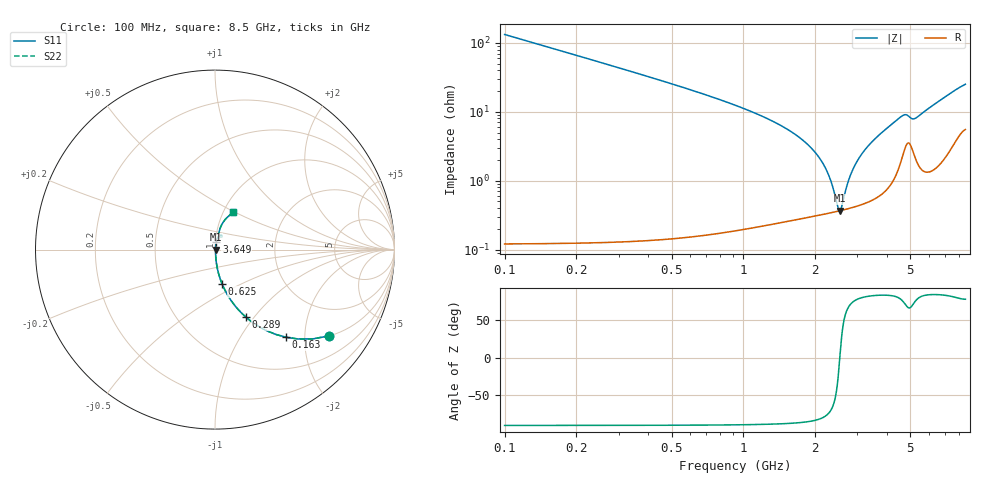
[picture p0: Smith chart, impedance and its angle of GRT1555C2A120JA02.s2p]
!Murata Part Number: GRT1555C2A120JA02
!These Parameters are Measured in Series Mode Connection
!Data Generated on Jun 19, 2026
!  o--ll--o
!Port1  Port2
!  o------o
!Operation Temp=25[degC], DC Bias Voltage=0[V]
!Freq. Start=100[MHz] Stop=9[GHz] 401[Steps]
# Hz S RI R 50
!Freq.(Hz) S11(Real) S11(Imag) S21(Real) S21(Imag) S12(Real) S12(Imag) S22(Real) S22(Imag)
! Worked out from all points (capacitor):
!   401 points, 100 MHz to 8.5 GHz, reference 50 ohm
!   read as one part in series: C = 12 pF near 142 MHz
!   lowest |Z| = 367 mohm at 2.536 GHz (marker M1)
!   series resonance near 2.532 GHz, so ESL is about 330 pH
!   S11 on the Smith chart (normalised r, x): 100 MHz: 1.00, -2.65; 163 MHz: 1.00, -1.62; 289 MHz: 1.00, -0.91; 625 MHz: 1.00, -0.40; 3.649 GHz: 1.01, +0.09; 8.5 GHz: 1.11, +0.49
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1e8  0.6367 -0.4805  0.3633 0.4805  0.3633 0.4805  0.6367 -0.4805
1.63e8  0.3965 -0.4884  0.6035 0.4884  0.6035 0.4884  0.3965 -0.4884
2.89e8  0.1709 -0.375  0.8291 0.375  0.8291 0.375  0.1709 -0.375
4.15e8  0.0892 -0.2829  0.9108 0.2829  0.9108 0.2829  0.0892 -0.2829
6.25e8  0.0396 -0.1911  0.9604 0.1911  0.9604 0.1911  0.0396 -0.1911
1.507e9  0.00578 -0.0568  0.9942 0.0568  0.9942 0.0568  0.00578 -0.0568
1.885e9  0.00395 -0.0317  0.996 0.0317  0.996 0.0317  0.00395 -0.0317
2.137e9  0.00354 -0.0182  0.9965 0.0182  0.9965 0.0182  0.00354 -0.0182
2.284e9  0.00349 -0.0111  0.9965 0.0111  0.9965 0.0111  0.00349 -0.0111
2.473e9  0.00359 -0.00256  0.9964 0.00256  0.9964 0.00256  0.00359 -0.00256
2.536e9  0.00365 0.000155  0.9963 -0.000155  0.9963 -0.000155  0.00365 0.000155
2.578e9  0.00371 0.00193  0.9963 -0.00193  0.9963 -0.00193  0.00371 0.00193
2.746e9  0.00399 0.00884  0.996 -0.00884  0.996 -0.00884  0.00399 0.00884
2.914e9  0.00438 0.0155  0.9956 -0.0155  0.9956 -0.0155  0.00438 0.0155
3.208e9  0.00534 0.0267  0.9947 -0.0267  0.9947 -0.0267  0.00534 0.0267
3.649e9  0.00762 0.0432  0.9924 -0.0432  0.9924 -0.0432  0.00762 0.0432
4.3e9  0.0157 0.069  0.9843 -0.069  0.9843 -0.069  0.0157 0.069
4.72e9  0.0337 0.0809  0.9663 -0.0809  0.9663 -0.0809  0.0337 0.0809
5.182e9  0.0286 0.0716  0.9714 -0.0716  0.9714 -0.0716  0.0286 0.0716
5.707e9  0.0228 0.0956  0.9772 -0.0956  0.9772 -0.0956  0.0228 0.0956
7.114e9  0.0491 0.1579  0.9509 -0.1579  0.9509 -0.1579  0.0491 0.1579
8.5e9  0.1008 0.2086  0.8992 -0.2086  0.8992 -0.2086  0.1008 0.2086
